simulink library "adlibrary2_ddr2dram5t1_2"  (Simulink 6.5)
undefined symbols (not defined in the file or in its folder): Bit, Black, blackbox2, blue, Box, ddr2sdram5t1_config, gcbh, Inactive, Location, Lower, VER_STRING_GOES_HERE, white, Width, xbsIndex_r4, xlBlockLoadCallback
libraries: xbsIndex_r4 x38, adlibrary2_ddr2dram5t1_2 x1

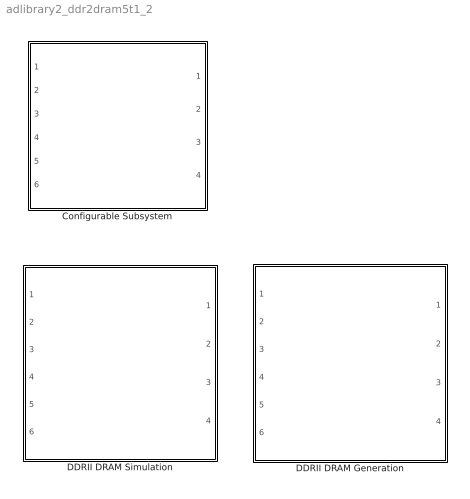
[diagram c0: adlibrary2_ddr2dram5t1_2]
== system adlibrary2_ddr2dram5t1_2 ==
  Configurable Subsystem : Subsystem  Tag=configX  BlockChoice=DDRII DRAM Simulation
  DDRII DRAM Generation : Subsystem
  DDRII DRAM Simulation : Subsystem

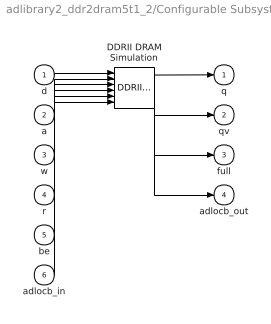
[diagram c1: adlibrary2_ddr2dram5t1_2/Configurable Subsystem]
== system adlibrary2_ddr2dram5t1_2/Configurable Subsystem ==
  d : Inport
  a : Inport  Port=2
  w : Inport  Port=3
  r : Inport  Port=4
  be : Inport  Port=5
  adlocb_in : Inport  Port=6
  DDRII DRAM Simulation : adlibrary2_ddr2dram5t1_2/DDRII DRAM Simulation  SystemSampleTime=-1
  q : Outport
  qv : Outport  Port=2
  full : Outport  Port=3
  adlocb_out : Outport  Port=4
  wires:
  d/1 -> DDRII DRAM Simulation/1
  a/1 -> DDRII DRAM Simulation/2
  w/1 -> DDRII DRAM Simulation/3
  r/1 -> DDRII DRAM Simulation/4
  be/1 -> DDRII DRAM Simulation/5
  adlocb_in/1 -> DDRII DRAM Simulation/6
  DDRII DRAM Simulation/1 -> q/1
  DDRII DRAM Simulation/2 -> qv/1
  DDRII DRAM Simulation/3 -> full/1
  DDRII DRAM Simulation/4 -> adlocb_out/1

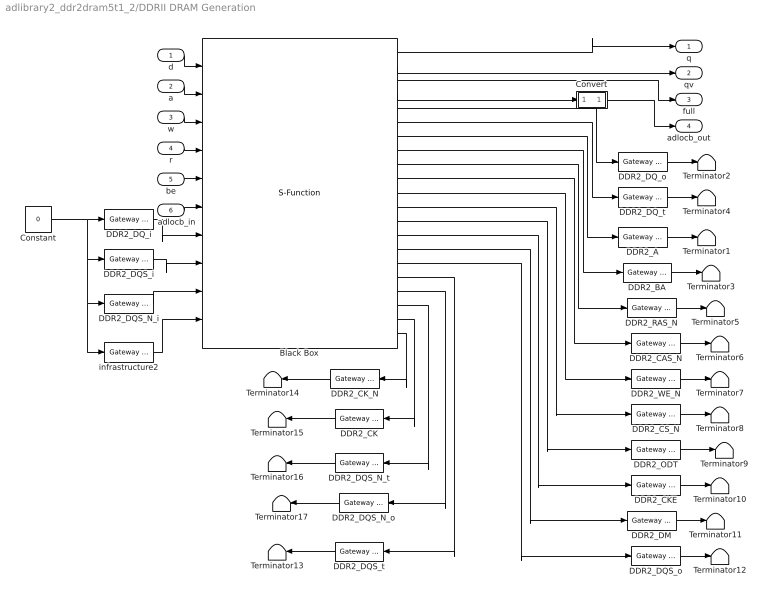
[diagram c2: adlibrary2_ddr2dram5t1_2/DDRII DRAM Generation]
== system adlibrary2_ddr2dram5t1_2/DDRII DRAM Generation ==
  d : Inport
  a : Inport  Port=2
  w : Inport  Port=3
  r : Inport  Port=4
  be : Inport  Port=5
  adlocb_in : Inport  Port=6
  Black Box : S-Function  AncestorBlock=xbsIndex_r4/Black Box  LoadFcn=xlBlockLoadCallback(gcbh);  FunctionName=sysgen  Parameters=ptable_  mask(Xilinx Black Box Block){infoedit=Incorporates black box HDL and simulation model into a System Generator design.<P><P>You must supply a Black Box with certain information about the HDL component you would like to bring into System Generator. This information is provided through a Matlab function.<P><P>When "Simulation mode" is set to "Inactive", you will typically want to provide a separate simulation model by using a Simulation 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, init_code=ddr2sdram5t1_config, sim_method=Inactive, sim_method_sgadvanced=, engine_block=, xl_use_area=off, xl_use_area_sgadvanced=, xl_area=[0,0,0,0,0,0,0], block_version=VER_STRING_GOES_HERE, has_advanced_control=0, sggui_pos=20,20,356,367, block_type=blackbox2, sg_icon_stat=220,350,10,21,white,blue,0,82d65d38, sg_mask_display=fprintf('','COMMENT: begin icon graphics '); patch([0 220 220 0 ],[0 0 350 350 ],[0.77 0.82 0.91]); patch([52 15 66 15 52 110 126 142 204 155 108 74 126 74 108 155 204 142 126 110 52 ],[89 126 177 228 265 265 249 265 265 216 263 229 177 125 91 138 89 89 105 89 89 ],[0.98 0.96 0.92]); plot([0 0 220 220 0 ],[0 350 350 0 0 ]); fprintf('','COMMENT: end icon graphics');  fprintf('','COMMENT: begin icon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, sg_list_contents=, adlocb_devid=1}
      mask prompts: infoedit ""; init_code "Block configuration m-function"; sim_method "Simulation mode"; engine_block "HDL co-simulator to use  (specify helper block by name)"; xl_use_area "Define FPGA area for resource estimation"; xl_area "FPGA area [slices, FFs, BRAMs, LUTs, IOBs, emb. mults, TBUFs]"; block_version ""; has_advanced_control ""; sggui_pos ""; block_type ""; sg_icon_stat ""; sg_mask_display ""; sg_list_contents ""; adlocb_devid "ADLOCB DEV ID"
      mask help: Incorporates black box HDL and simulation model into a System Generator design. You must supply a Black Box with certain information about the HDL component you would like to bring into System Generator. This information is provided through a Matlab function. When "Simulation mode" is set to "Inactive", you will typically want to provide a separate simulation model by using a Simulation Multiplexer. When "Simulation mode" is set to "External co-simulator", you must include a ModelSim block in the design.
      mask init:
      | xlMungeMaskParams;
      | 
      | mdlPath = xlGetMdlDir(bdroot);
      | 
      | refBlk = get_param(gcb,'referenceBlock');
      | if (isempty(refBlk) | strncmp(refBlk,'xbsIndex',8))
      | srcPath = mdlPath;
      | else
      | srcPath = xlPathToReference;
      | if (isempty(srcPath))
      | srcPath = mdlPath;
      | end
      | end
      | 
      | if (sim_method==3)
      | validEngineBlock = 0;
      | try
      | engineBlock = xlBlockNameRelPath(get_param(gcb,'Parent'),engine_block);
      | catch
      | engineBlock = '//';
      | end
      | try 
      | engineWorkDir = get_param(engineBlock,'dir');
      | validEngineBlock = 1;
      | engine_handle = get_param(engineBlock,'Handle');
      | catch
      | end
      | end
      | 
      | % build black box config function
      | block_config = ['sysgen:black_box_config:' init_code];
      | 
      | serialized_declarations = '{''engine_handle''=>''Double'',''sim_method''=>''Int'',''validEngineBlock''=>''Int'',''engineWorkDir''=>''String'',''engine_block''=>''String'',''init_code''=>''String'',''mdlPath''=>''String'',''srcPath''=>''String'',''block_config''=>''String'',}';
      | ptable_ = xlblockprep(get_param(gcb, 'MaskWSVariables'));
  Constant : Constant  Value=0  OutDataType=sfix(16)  ConRadixGroup=Use specified scaling  OutScaling=2^0  SampleTime=inf  FramePeriod=inf
  Convert : Subsystem
  DDR2_A : xbsIndex_r4/Gateway Out  hdl_port=on  timing_constraint=None  locs_specified=off  LOCs={}  block_type=gatewayout
  DDR2_BA : xbsIndex_r4/Gateway Out  hdl_port=on  timing_constraint=None  locs_specified=off  LOCs={}  block_type=gatewayout
  DDR2_CAS_N : xbsIndex_r4/Gateway Out  hdl_port=on  timing_constraint=None  locs_specified=off  LOCs={}  block_type=gatewayout
  DDR2_CK : xbsIndex_r4/Gateway Out  Orientation=left  hdl_port=on  timing_constraint=None  locs_specified=off  LOCs={}  block_type=gatewayout
  DDR2_CKE : xbsIndex_r4/Gateway Out  hdl_port=on  timing_constraint=None  locs_specified=off  LOCs={}  block_type=gatewayout
  DDR2_CK_N : xbsIndex_r4/Gateway Out  Orientation=left  hdl_port=on  timing_constraint=None  locs_specified=off  LOCs={}  block_type=gatewayout
  DDR2_CS_N : xbsIndex_r4/Gateway Out  hdl_port=on  timing_constraint=None  locs_specified=off  LOCs={}  block_type=gatewayout
  DDR2_DM : xbsIndex_r4/Gateway Out  hdl_port=on  timing_constraint=None  locs_specified=off  LOCs={}  block_type=gatewayout
  DDR2_DQS_N_i : xbsIndex_r4/Gateway In  arith_type=Unsigned  n_bits=4  bin_pt=0  quantization="Round  (unbiased: +/- Inf)"  overflow=Saturate  period=ad_get_simulink_period  dbl_ovrd=off  timing_constraint=None  locs_specified=off  LOCs={}  block_type=gatewayin
  DDR2_DQS_N_o : xbsIndex_r4/Gateway Out  Orientation=left  hdl_port=on  timing_constraint=None  locs_specified=off  LOCs={}  block_type=gatewayout
  DDR2_DQS_N_t : xbsIndex_r4/Gateway Out  Orientation=left  hdl_port=on  timing_constraint=None  locs_specified=off  LOCs={}  block_type=gatewayout
  DDR2_DQS_i : xbsIndex_r4/Gateway In  arith_type=Unsigned  n_bits=4  bin_pt=0  quantization="Round  (unbiased: +/- Inf)"  overflow=Saturate  period=ad_get_simulink_period  dbl_ovrd=off  timing_constraint=None  locs_specified=off  LOCs={}  block_type=gatewayin
  DDR2_DQS_o : xbsIndex_r4/Gateway Out  hdl_port=on  timing_constraint=None  locs_specified=off  LOCs={}  block_type=gatewayout
  DDR2_DQS_t : xbsIndex_r4/Gateway Out  Orientation=left  hdl_port=on  timing_constraint=None  locs_specified=off  LOCs={}  block_type=gatewayout
  DDR2_DQ_i : xbsIndex_r4/Gateway In  arith_type=Unsigned  n_bits=32  bin_pt=0  quantization="Round  (unbiased: +/- Inf)"  overflow=Saturate  period=ad_get_simulink_period  dbl_ovrd=off  timing_constraint=None  locs_specified=off  LOCs={}  block_type=gatewayin
  DDR2_DQ_o : xbsIndex_r4/Gateway Out  hdl_port=on  timing_constraint=None  locs_specified=off  LOCs={}  block_type=gatewayout
  DDR2_DQ_t : xbsIndex_r4/Gateway Out  hdl_port=on  timing_constraint=None  locs_specified=off  LOCs={}  block_type=gatewayout
  DDR2_ODT : xbsIndex_r4/Gateway Out  hdl_port=on  timing_constraint=None  locs_specified=off  LOCs={}  block_type=gatewayout
  DDR2_RAS_N : xbsIndex_r4/Gateway Out  hdl_port=on  timing_constraint=None  locs_specified=off  LOCs={}  block_type=gatewayout
  DDR2_WE_N : xbsIndex_r4/Gateway Out  hdl_port=on  timing_constraint=None  locs_specified=off  LOCs={}  block_type=gatewayout
  Terminator{1..17} (17 alike) : Terminator
  infrastructure2 : xbsIndex_r4/Gateway In  arith_type=Unsigned  n_bits=11  bin_pt=0  quantization="Round  (unbiased: +/- Inf)"  overflow=Saturate  period=ad_get_simulink_period  dbl_ovrd=off  timing_constraint=None  locs_specified=off  LOCs={}  block_type=gatewayin
  q : Outport
  qv : Outport  Port=2
  full : Outport  Port=3
  adlocb_out : Outport  Port=4
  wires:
  DDR2_DQ_o/1 -> Terminator2/1
  Constant/1 -> DDR2_DQ_i/1, DDR2_DQS_N_i/1, infrastructure2/1, DDR2_DQS_i/1
  d/1 -> Black Box/1
  a/1 -> Black Box/2
  w/1 -> Black Box/3
  r/1 -> Black Box/4
  be/1 -> Black Box/5
  adlocb_in/1 -> Black Box/6
  DDR2_DQ_i/1 -> Black Box/7
  DDR2_DQS_i/1 -> Black Box/8
  DDR2_DQS_N_i/1 -> Black Box/9
  infrastructure2/1 -> Black Box/10
  Black Box/1 -> q/1
  Black Box/2 -> qv/1
  Black Box/3 -> full/1
  Black Box/4 -> Convert/1(in0)
  Black Box/5 -> DDR2_DQ_o/1
  DDR2_DQ_t/1 -> Terminator4/1
  Black Box/6 -> DDR2_DQ_t/1
  DDR2_A/1 -> Terminator1/1
  Black Box/7 -> DDR2_A/1
  DDR2_BA/1 -> Terminator3/1
  Convert/1(out0) -> adlocb_out/1
  Black Box/8 -> DDR2_BA/1
  DDR2_RAS_N/1 -> Terminator5/1
  Black Box/9 -> DDR2_RAS_N/1
  DDR2_CAS_N/1 -> Terminator6/1
  Black Box/10 -> DDR2_CAS_N/1
  Black Box/11 -> DDR2_WE_N/1
  DDR2_WE_N/1 -> Terminator7/1
  DDR2_CS_N/1 -> Terminator8/1
  DDR2_ODT/1 -> Terminator9/1
  DDR2_CKE/1 -> Terminator10/1
  DDR2_DM/1 -> Terminator11/1
  DDR2_DQS_o/1 -> Terminator12/1
  DDR2_CK_N/1 -> Terminator14/1
  Black Box/12 -> DDR2_CS_N/1
  Black Box/13 -> DDR2_ODT/1
  Black Box/14 -> DDR2_CKE/1
  Black Box/15 -> DDR2_DM/1
  Black Box/16 -> DDR2_DQS_o/1
  DDR2_CK/1 -> Terminator15/1
  DDR2_DQS_N_t/1 -> Terminator16/1
  DDR2_DQS_N_o/1 -> Terminator17/1
  DDR2_DQS_t/1 -> Terminator13/1
  Black Box/21 -> DDR2_CK_N/1
  Black Box/20 -> DDR2_CK/1
  Black Box/19 -> DDR2_DQS_N_t/1
  Black Box/18 -> DDR2_DQS_N_o/1
  Black Box/17 -> DDR2_DQS_t/1

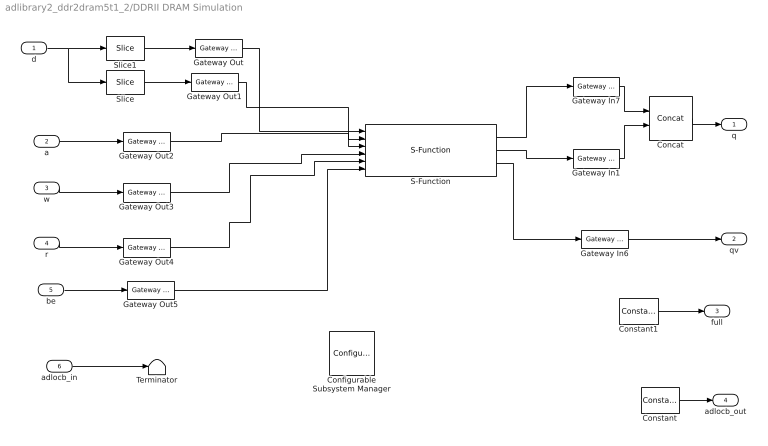
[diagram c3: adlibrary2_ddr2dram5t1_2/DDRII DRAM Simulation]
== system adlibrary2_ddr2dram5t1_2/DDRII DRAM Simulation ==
  d : Inport
  a : Inport  Port=2
  w : Inport  Port=3
  r : Inport  Port=4
  be : Inport  Port=5
  adlocb_in : Inport  Port=6
  Concat : xbsIndex_r4/Concat  num_inputs=2  dbl_ovrd=off  block_type=concat
  Configurable Subsystem Manager : xbsIndex_r4/Configurable Subsystem Manager  Tag=xcfgMgr  block_type=configsubsys
  Constant : xbsIndex_r4/Constant  arith_type=Signed (2's comp)  const=0  n_bits=66  bin_pt=0  explicit_period=on  period=ad_get_simulink_period  equ=P=C  opselect=C  inp2=PCIN>>17  opr=+  inp1=P  carry=CIN  dbl_ovrd=off  block_type=constant
  Constant1 : xbsIndex_r4/Constant  arith_type=Boolean  const=0  n_bits=66  bin_pt=0  explicit_period=on  period=ad_get_simulink_period  equ=P=C  opselect=C  inp2=PCIN>>17  opr=+  inp1=P  carry=CIN  dbl_ovrd=off  block_type=constant
  Gateway In1 : xbsIndex_r4/Gateway In  arith_type=Unsigned  n_bits=32  bin_pt=0  quantization="Round  (unbiased: +/- Inf)"  overflow=Saturate  period=ad_get_simulink_period  dbl_ovrd=on  timing_constraint=None  locs_specified=off  LOCs={}  block_type=gatewayin
  Gateway In6 : xbsIndex_r4/Gateway In  arith_type=Boolean  n_bits=1  bin_pt=0  quantization="Round  (unbiased: +/- Inf)"  overflow=Saturate  period=ad_get_simulink_period  dbl_ovrd=on  timing_constraint=None  locs_specified=off  LOCs={}  block_type=gatewayin
  Gateway In7 : xbsIndex_r4/Gateway In  arith_type=Unsigned  n_bits=32  bin_pt=0  quantization="Round  (unbiased: +/- Inf)"  overflow=Saturate  period=ad_get_simulink_period  dbl_ovrd=on  timing_constraint=None  locs_specified=off  LOCs={}  block_type=gatewayin
  Gateway Out{,1..5} (6 alike) : xbsIndex_r4/Gateway Out  hdl_port=off  timing_constraint=None  locs_specified=off  LOCs={}  block_type=gatewayout
  S-Function : S-Function  FunctionName=ddr2dram  Parameters=1
  Slice : xbsIndex_r4/Slice  nbits=32  boolean_output=off  mode=Lower Bit Location + Width  bit1=0  base1=MSB of Input  bit0=0  base0=LSB of Input  dbl_ovrd=off  block_type=slice
  Slice1 : xbsIndex_r4/Slice  nbits=32  boolean_output=off  mode=Lower Bit Location + Width  bit1=0  base1=MSB of Input  bit0=32  base0=LSB of Input  dbl_ovrd=off  block_type=slice
  Terminator : Terminator
  q : Outport
  qv : Outport  Port=2
  full : Outport  Port=3
  adlocb_out : Outport  Port=4
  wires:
  Concat/1 -> q/1
  Gateway In1/1 -> Concat/2
  Gateway In7/1 -> Concat/1
  d/1 -> Slice/1, Slice1/1
  Slice/1 -> Gateway Out1/1
  Slice1/1 -> Gateway Out/1
  Gateway Out5/1 -> S-Function/6
  be/1 -> Gateway Out5/1
  S-Function/3 -> Gateway In6/1
  Gateway In6/1 -> qv/1
  S-Function/2 -> Gateway In1/1
  Gateway Out4/1 -> S-Function/5
  r/1 -> Gateway Out4/1
  Gateway Out3/1 -> S-Function/4
  Gateway Out2/1 -> S-Function/3
  Gateway Out1/1 -> S-Function/2
  Gateway Out/1 -> S-Function/1
  S-Function/1 -> Gateway In7/1
  w/1 -> Gateway Out3/1
  a/1 -> Gateway Out2/1
  Constant/1 -> adlocb_out/1
  adlocb_in/1 -> Terminator/1
  Constant1/1 -> full/1

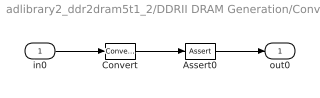
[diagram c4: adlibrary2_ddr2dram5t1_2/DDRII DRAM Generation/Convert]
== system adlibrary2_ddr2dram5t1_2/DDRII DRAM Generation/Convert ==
  in0 : Inport
  Assert0 : xbsIndex_r4/Assert  assert_type=off  type_source=Explicitly  arith_type="Signed  (2's comp)"  n_bits=16  bin_pt=14  assert_rate=on  rate_source=Explicitly  period=ad_get_simulink_period  output_port=on  block_type=assert
  Convert : xbsIndex_r4/Convert  arith_type=Unsigned  n_bits=66  bin_pt=0  quantization=Truncate  overflow=Wrap  latency=0  dbl_ovrd=off  pipeline=off  block_type=convert
  out0 : Outport
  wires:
  in0/1 -> Convert/1
  Convert/1 -> Assert0/1
  Assert0/1 -> out0/1
